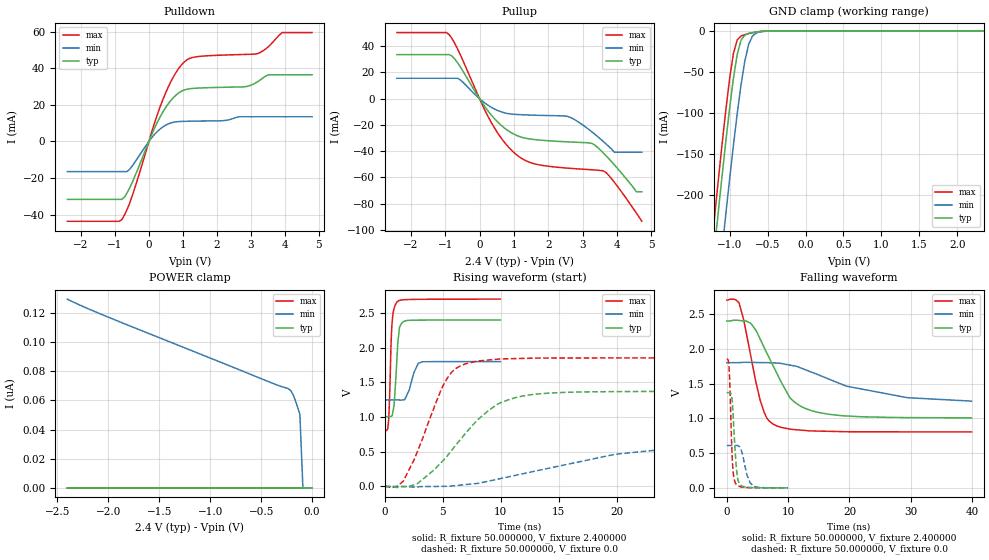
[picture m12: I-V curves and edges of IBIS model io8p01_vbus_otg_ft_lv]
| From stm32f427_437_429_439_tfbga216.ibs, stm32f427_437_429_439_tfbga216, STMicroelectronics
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|   Model io8p01_vbus_otg_ft_lv
[Model]  io8p01_vbus_otg_ft_lv
Model_type I/O
Polarity   Non-Inverting
Enable   Active-Low
Vinl =   0.720000V
Vinh =   1.680000V
Vmeas =  1.200000V
Cref =   50.000000pF
Rref =   100.000000M
Vref =   0.0V
C_comp   3.193600pF   3.100000pF   3.332100pF
[Temperature Range]   25.000000   0.125000k   -40.000000
[Pullup Reference]   2.400000V   1.800000V   2.700000V
[Pulldown Reference]   0.0V   0.0V   0.0V
[POWER Clamp Reference]   2.400000V   1.800000V   2.700000V
[GND Clamp Reference]   0.0V   0.0V   0.0V
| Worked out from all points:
|   slope of the pulldown table from 0 to 0.36 V, typ, clamps not added: 25 ohm
|   slope of the pullup table from 0 to 0.36 V, typ, clamps not added: 27.7 ohm
|   GND clamp passes 1 mA (typ) near -0.61 V on its own axis
|   rising waveform, R_fixture 50.000000, V_fixture 2.400000: 20-80 % time 310ps typ, 630ps min, 224ps max; typ from 1.01 V to 2.4 V
|   rising waveform, R_fixture 50.000000, V_fixture 0.0: 20-80 % time 4.51ns typ, 11ns min, 2.64ns max; typ from 0 V to 1.37 V
|   falling waveform, R_fixture 50.000000, V_fixture 2.400000: 20-80 % time 4.85ns typ, 12.7ns min, 2.75ns max; typ from 2.4 V to 1.01 V
|   falling waveform, R_fixture 50.000000, V_fixture 0.0: 20-80 % time 575ps typ, 1.04ns min, 435ps max; typ from 1.37 V to 0 V
[Pulldown]
|Voltage   I(typ)   I(min)   I(max)
-2.4V     -31.69mA   -16.5mA    -43.66mA
-800mV    -31.69mA   -16.5mA    -42.82mA
-480mV    -21.96mA   -13.17mA   -29.19mA
80mV      3.63mA     1.966mA    5.014mA
480mV     18.16mA    8.738mA    26.02mA
800mV     25.38mA    10.72mA    37.77mA
1.12V     28.53mA    11.02mA    44.6mA
2.8V      29.84mA    13.49mA    47.53mA
3.2V      32.65mA    13.49mA    48.05mA
3.52V     36.43mA    13.49mA    51.84mA
3.92V     36.43mA    13.49mA    59.49mA
4.8V      36.43mA    13.49mA    59.49mA
[Pullup]
|Voltage   I(typ)   I(min)   I(max)
-2.4V     33.57mA    15.56mA    50.37mA
-960mV    33.57mA    15.56mA    50.37mA
-560mV    24.29mA    14.3mA     33.55mA
320mV     -11.75mA   -6.207mA   -17.08mA
960mV     -26.47mA   -11.82mA   -40.02mA
1.52V     -30.88mA   -12.51mA   -49.05mA
2.56V     -32.88mA   -13.49mA   -52.9mA
3.28V     -34.19mA   -25.52mA   -54.18mA
3.6V      -41.31mA   -32.61mA   -54.99mA
3.92V     -50.32mA   -40.8mA    -63.62mA
4.56V     -70.9mA    -40.8mA    -87.08mA
4.72V     -70.9mA    -40.8mA    -93.4mA
[GND_clamp]
|Voltage   I(typ)   I(min)   I(max)
-2.4V     -1.425A    -1.509A    -1.394A
-1.25V    -311.3mA   -401.9mA   -273.4mA
-1.2V     -265.5mA   -356.1mA   -227.3mA
-1.15V    -220.5mA   -310.9mA   -182mA
-1.1V     -176.4mA   -266.2mA   -138mA
-1.05V    -133.9mA   -222.5mA   -96.06mA
-950mV    -57.51mA   -139mA     -27.35mA
-900mV    -28.55mA   -100.5mA   -11.03mA
-850mV    -11.33mA   -65.67mA   -6.322mA
-750mV    -3.069mA   -16.69mA   -3.425mA
-600mV    -864.6uA   -1.294mA   -852.2uA
2.35V     0A         0A         0A
[POWER_clamp]
|Voltage   I(typ)   I(min)   I(max)
-2.4V     0A         129.4nA    0A
-1.98V    0A         116.5nA    0A
-390mV    0A         71.78nA    0A
-240mV    0A         68.22nA    0A
-210mV    0A         66.81nA    0A
-180mV    0A         62.95nA    0A
-120mV    0A         50.47nA    0A
-90mV     0A         0A         0A
0V        0A         0A         0A
[Ramp]
| variable   typ   min   max
dV/dt_r  0.82218/4.50373n   0.36607/11.19903n   1.11102/2.63513n
dV/dt_f  0.83652/4.85156n   0.32286/13.23292n   1.13834/2.75525n
R_load = 50.000000
[Rising Waveform]
R_fixture= 50.000000
V_fixture= 2.400000
V_fixture_min= 1.800000
V_fixture_max= 2.700000
|time   V(typ)   V(min)   V(max)
0s        1.006V     1.247V     804.6mV
340.3ps   1.006V     1.247V     971.5mV
560.6ps   1.012V     1.247V     2.143V
640.6ps   1.024V     1.247V     2.378V
800.8ps   1.167V     1.247V     2.566V
1.041ns   1.825V     1.247V     2.656V
1.261ns   2.28V      1.246V     2.681V
1.682ns   2.381V     1.249V     2.691V
2.903ns   2.397V     1.776V     2.697V
9.97ns    2.4V       1.8V       2.7V
[Rising Waveform]
R_fixture= 50.000000
V_fixture= 0.0
V_fixture_min= 0.0
V_fixture_max= 0.0
|time   V(typ)   V(min)   V(max)
0s        177.7uV    73.62uV    454.6uV
1.602ns   -2.594mV   -134.3uV   78.46mV
2.803ns   39.13mV    -5.997mV   498.4mV
5.045ns   375.6mV    1.766mV    1.46V
5.926ns   554.3mV    9.804mV    1.672V
7.047ns   783.4mV    28.33mV    1.772V
9.69ns    1.182V     103.3mV    1.834V
12.89ns   1.327V     218.7mV    1.849V
26.51ns   1.37V      576mV      1.852V
39.88ns   1.37V      609mV      1.852V
[Falling Waveform]
R_fixture= 50.000000
V_fixture= 2.400000
V_fixture_min= 1.800000
V_fixture_max= 2.700000
|time   V(typ)   V(min)   V(max)
0s        2.4V       1.8V       2.7V
2.002ns   2.407V     1.801V     2.661V
3.924ns   2.365V     1.805V     1.895V
5.445ns   2.14V      1.801V     1.261V
6.567ns   1.932V     1.8V       999.5mV
7.768ns   1.718V     1.796V     907mV
10.33ns   1.291V     1.764V     844.2mV
14.01ns   1.105V     1.657V     818.2mV
29.39ns   1.01V      1.297V     805mV
39.88ns   1.006V     1.247V     804.6mV
[Falling Waveform]
R_fixture= 50.000000
V_fixture= 0.0
V_fixture_min= 0.0
V_fixture_max= 0.0
|time   V(typ)   V(min)   V(max)
0s        1.37V      609mV      1.852V
380.4ps   1.37V      609.1mV    1.725V
860.9ps   1.273V     608.9mV    504.9mV
1.061ns   1.019V     608.6mV    213.5mV
1.401ns   488.7mV    608.8mV    73.88mV
1.742ns   157.8mV    609.7mV    35.08mV
2.342ns   33.79mV    546.6mV    13.71mV
3.343ns   8.003mV    173.8mV    4.09mV
4.464ns   2.726mV    18.5mV     1.536mV
9.97ns    177.7uV    73.62uV    454.6uV
